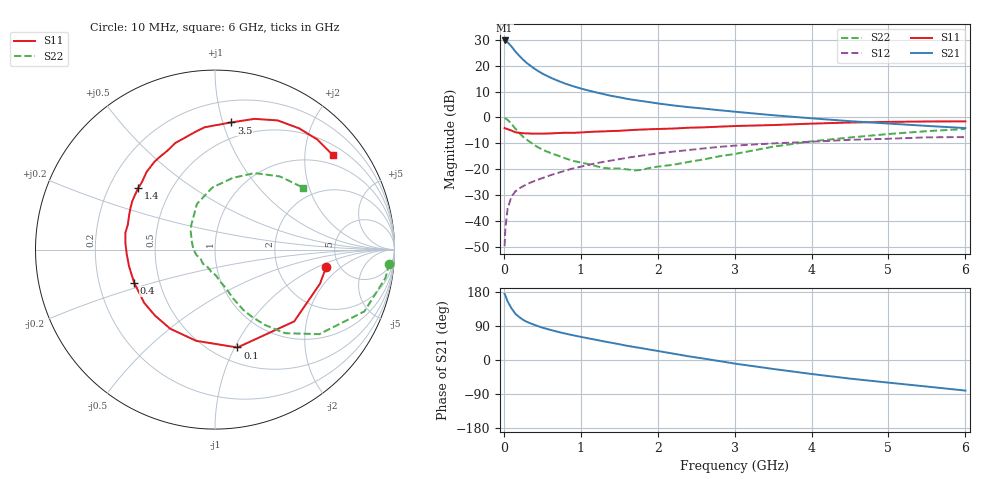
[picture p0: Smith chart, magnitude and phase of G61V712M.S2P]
! SIEMENS Small Signal Semiconductors
! BFG193
! Si NPN RF Bipolar Junction Transistor in SOT223
! VCE = 1.75 V  IC = 12 mA
! Common Emitter S-Parameters:  August  1996
# GHz  S  MA  R  50
!  f  S11  S21  S12  S22
! GHz  MAG  ANG  MAG  ANG  MAG  ANG  MAG  ANG
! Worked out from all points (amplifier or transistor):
!   36 points, 10 MHz to 6 GHz, reference 50 ohm
!   highest |S21| = 29.7 dB at 10 MHz (marker M1)
!   |S21| within 3 dB of that: start of sweep to 117.1 MHz
!   unconditionally stable (mu >= 1): 813.8 MHz to 2.712 GHz
!   at 250 MHz: K = 0.60, MSG = 24.4 dB, |S12| = -26.5 dB
!   at 1.4 GHz: K = 1.07, MAG = 10.9 dB, |S12| = -16.6 dB
!   at 6 GHz: K = 0.92, MSG = 1.7 dB, |S12| = -7.6 dB
!   S11 on the Smith chart (normalised r, x): 10 MHz: 3.93, -1.26; 100 MHz: 0.65, -1.03; 400 MHz: 0.36, -0.17; 1.4 GHz: 0.32, +0.32; 3.5 GHz: 0.37, +1.07; 6 GHz: 0.73, +2.65
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0.01  0.6269 -8.9  30.57 174.5  0.0033 89.5  0.9744 -4.6
0.02  0.6151 -18.0  30.22 169.8  0.0074 82.1  0.9625 -9.5
0.05  0.5956 -42.2  28.14 154.2  0.0177 72.8  0.9005 -22.5
0.1  0.5595 -77.1  23.33 136.2  0.0301 60.7  0.7485 -39.0
0.15  0.5189 -101.7  18.73 122.0  0.0375 54.7  0.6079 -50.0
0.2  0.5066 -119.5  15.53 113.2  0.0429 51.9  0.5061 -56.3
0.25  0.4968 -132.5  13.03 106.0  0.0472 50.4  0.4246 -61.4
0.3  0.4936 -143.1  11.19 100.6  0.052 50.2  0.3719 -64.8
0.4  0.4868 -157.7  8.679 92.5  0.0598 50.3  0.2908 -69.6
0.5  0.4879 -169.0  7.025 85.4  0.0677 50.9  0.2398 -72.8
0.6  0.4925 -177.1  5.933 79.8  0.0765 51.1  0.2089 -76.0
0.7  0.5003 175.9  5.125 74.5  0.0852 51.3  0.1848 -80.0
0.9  0.5052 164.0  4.012 65.3  0.1043 50.4  0.1459 -87.3
1.1  0.5247 154.0  3.309 57.1  0.1218 48.7  0.1263 -99.1
1.4  0.5481 141.4  2.607 45.5  0.1482 44.4  0.1035 -120.1
1.7  0.5769 131.3  2.17 34.1  0.1758 39.6  0.0952 -145.4
2.2  0.6118 115.6  1.709 16.9  0.2197 29.5  0.1222 175.8
2.8  0.6651 99.5  1.381 -2.8  0.271 16.6  0.1784 140.1
3.5  0.7144 82.7  1.105 -23.6  0.3165 0.0  0.2736 111.6
4.5  0.8001 64.1  0.849 -49.1  0.371 -19.6  0.4114 76.1
5.5  0.8374 47.1  0.688 -70.1  0.4142 -42.8  0.545 48.4
6  0.8414 38.9  0.625 -80.7  0.4184 -56.1  0.6004 35.1
